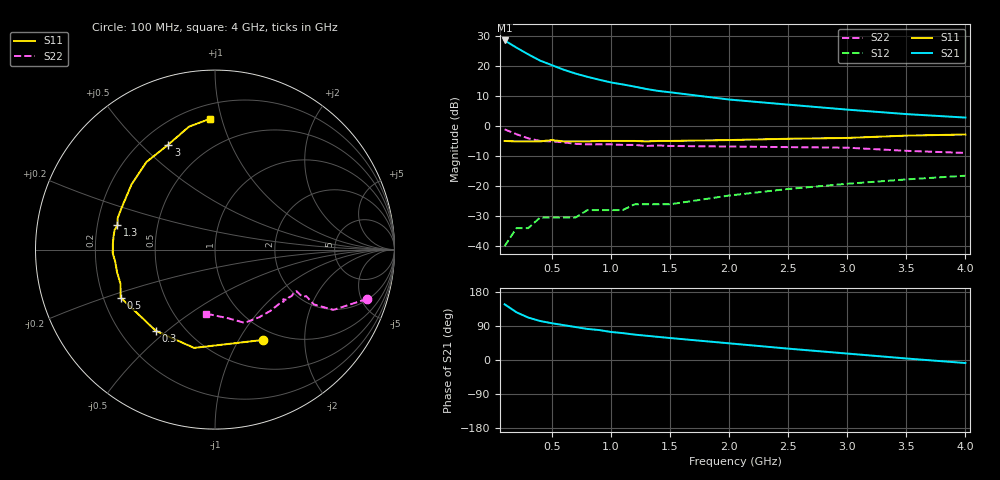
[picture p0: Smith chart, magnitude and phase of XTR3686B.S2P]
! HXTR-3686 Typical S-Parameters
! (Vce = 10 V, Ic = 15 mA)
# ghz s ma r 50
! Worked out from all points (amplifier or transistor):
!   20 points, 100 MHz to 4 GHz, reference 50 ohm
!   highest |S21| = 28.7 dB at 100 MHz (marker M1)
!   |S21| within 3 dB of that: start of sweep to 227.5 MHz
!   unconditionally stable (mu >= 1): 990 MHz to 1.172 GHz; 1.226 GHz to 2.732 GHz
!   at 400 MHz: K = 0.57, MSG = 26.2 dB, |S12| = -30.5 dB
!   at 1.1 GHz: K = 1.11, MAG = 18.9 dB, |S12| = -28.0 dB
!   at 4 GHz: K = 0.87, MSG = 9.7 dB, |S12| = -16.5 dB
!   S11 on the Smith chart (normalised r, x): 100 MHz: 0.85, -1.27; 300 MHz: 0.35, -0.46; 500 MHz: 0.27, -0.22; 1.3 GHz: 0.29, +0.11; 3 GHz: 0.31, +0.61; 4 GHz: 0.29, +0.92
0.1  0.57 -62.0  27.1 147.0  0.01 65.0  0.89 -18.0
0.2  0.56 -102.0  20.6 126.0  0.02 53.0  0.74 -27.0
0.3  0.56 -126.0  15.9 112.0  0.02 48.0  0.63 -29.0
0.4  0.56 -141.0  12.5 103.0  0.03 46.0  0.57 -27.0
0.5  0.59 -153.0  10.5 97.0  0.03 46.0  0.56 -28.0
0.6  0.56 -160.0  8.8 92.0  0.03 47.0  0.54 -28.0
0.7  0.56 -167.0  7.6 87.0  0.03 49.0  0.51 -27.0
0.8  0.56 -173.0  6.7 82.0  0.04 50.0  0.5 -29.0
0.9  0.57 -178.0  6 79.0  0.04 52.0  0.5 -29.0
1  0.57 177.0  5.4 74.0  0.04 53.0  0.5 -31.0
1.1  0.57 173.0  5 71.0  0.04 53.0  0.49 -33.0
1.2  0.57 169.0  4.6 67.0  0.05 54.0  0.49 -35.0
1.3  0.56 166.0  4.2 64.0  0.05 55.0  0.47 -36.0
1.4  0.57 162.0  3.9 61.0  0.05 55.0  0.48 -37.0
1.5  0.57 156.0  3.7 58.0  0.05 55.0  0.47 -39.0
2  0.59 142.0  2.8 44.0  0.07 55.0  0.46 -48.0
2.5  0.62 128.0  2.3 30.0  0.09 54.0  0.45 -57.0
3  0.64 114.0  1.9 17.0  0.11 50.0  0.44 -68.0
3.5  0.7 102.0  1.6 4.0  0.13 45.0  0.39 -79.0
4  0.73 92.0  1.4 -8.0  0.15 40.0  0.36 -98.0
